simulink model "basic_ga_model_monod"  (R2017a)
settings: Solver=ode45  StartTime=0  StopTime=30  MaxStep=0.001  RelTol=1e-6  AbsTol=1e-6  EnableMultiTasking=on
undefined symbols (not defined in the file or in its folder): GA0, K, K1, K2, K3, Kga, Muga, Mumax, O20, S0, X0

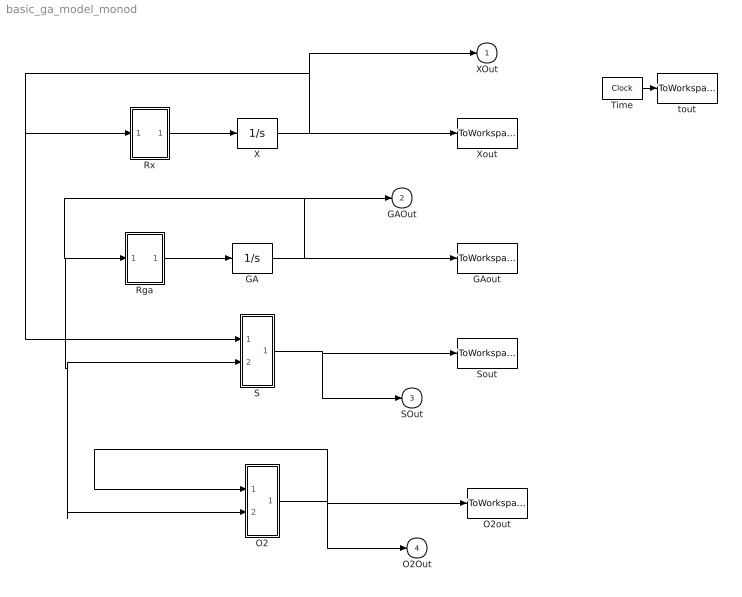
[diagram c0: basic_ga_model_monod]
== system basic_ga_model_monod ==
  GA : Integrator  InitialCondition=GA0  UpperSaturationLimit=1000  LowerSaturationLimit=0
  GAout : ToWorkspace  VariableName=GAout  SampleTime=-1
  O2 : Subsystem
  O2out : ToWorkspace  VariableName=O2out  SampleTime=-1
  Rga : Subsystem
  Rx : Subsystem
  S : Subsystem
  Sout : ToWorkspace  VariableName=Sout  SampleTime=-1
  Time : Clock
  X : Integrator  InitialCondition=X0  UpperSaturationLimit=1000  LowerSaturationLimit=0
  Xout : ToWorkspace  VariableName=Xout  SampleTime=-1
  tout : ToWorkspace  VariableName=tout  SampleTime=-1
  XOut : Outport
  GAOut : Outport  Port=2
  SOut : Outport  Port=3
  O2Out : Outport  Port=4
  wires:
  S/1(Sout) -> SOut/1, Sout/1
  Time/1 -> tout/1
  Rx/1(Rx) -> X/1
  Rga/1(Rga) -> GA/1
  GA/1 -> GAOut/1, O2/2(Rga), S/2(Rga), Rga/1(GA), GAout/1
  X/1 -> Xout/1, XOut/1, Rx/1(X), S/1(Rx)
  O2/1(O2out) -> O2/1(O2), O2Out/1, O2out/1

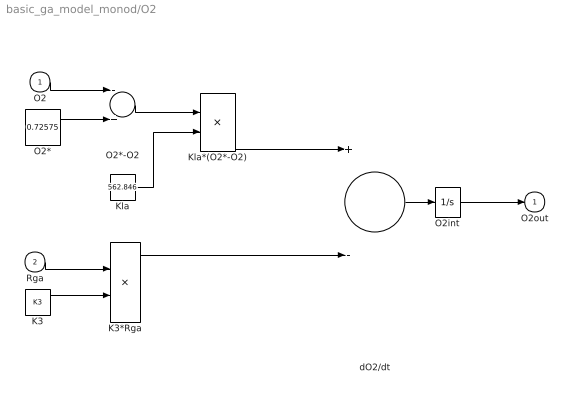
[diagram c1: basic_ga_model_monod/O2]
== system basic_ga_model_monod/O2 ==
  O2 : Inport
  Rga : Inport  Port=2
  K3 : Constant  Value=K3
  K3*Rga : Product
  Kla : Constant  Value=562.846
  Kla*(O2*-O2) : Product
  O2* : Constant  Value=0.72575
  O2*-O2 : Sum  Inputs=-+
  O2int : Integrator  InitialCondition=O20  UpperSaturationLimit=1000  LowerSaturationLimit=0
  dO2/dt : Sum  Inputs=+-
  O2out : Outport
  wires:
  O2int/1 -> O2out/1
  O2/1 -> O2*-O2/1
  K3*Rga/1 -> dO2/dt/2
  dO2/dt/1 -> O2int/1
  O2*/1 -> O2*-O2/2
  Rga/1 -> K3*Rga/1
  K3/1 -> K3*Rga/2
  O2*-O2/1 -> Kla*(O2*-O2)/1
  Kla/1 -> Kla*(O2*-O2)/2
  Kla*(O2*-O2)/1 -> dO2/dt/1

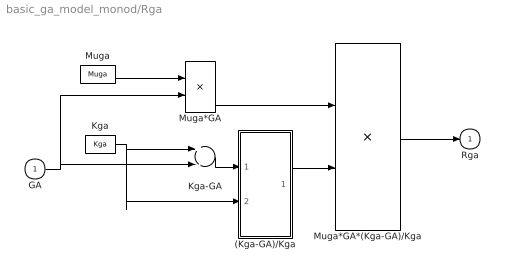
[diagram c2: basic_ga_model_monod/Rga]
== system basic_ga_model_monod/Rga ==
  GA : Inport
  (Kga-GA)/Kga : Subsystem
  Kga : Constant  Value=Kga
  Kga-GA : Sum  Inputs=+-
  Muga : Constant  Value=Muga
  Muga*GA : Product
  Muga*GA*(Kga-GA)/Kga : Product
  Rga : Outport
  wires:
  Muga*GA*(Kga-GA)/Kga/1 -> Rga/1
  Muga/1 -> Muga*GA/1
  Muga*GA/1 -> Muga*GA*(Kga-GA)/Kga/1
  GA/1 -> Kga-GA/2, Muga*GA/2
  Kga/1 -> (Kga-GA)/Kga/2(Ks+S), Kga-GA/1
  Kga-GA/1 -> (Kga-GA)/Kga/1(Mmax*S)
  (Kga-GA)/Kga/1(out_1) -> Muga*GA*(Kga-GA)/Kga/2

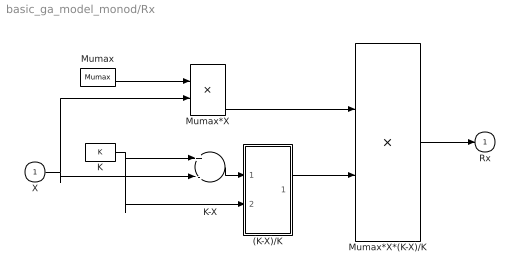
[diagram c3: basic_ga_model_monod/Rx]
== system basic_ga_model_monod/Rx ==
  X : Inport
  (K-X)/K : Subsystem
  K : Constant  Value=K
  K-X : Sum  Inputs=+-
  Mumax : Constant  Value=Mumax
  Mumax*X : Product
  Mumax*X*(K-X)/K : Product
  Rx : Outport
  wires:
  Mumax*X*(K-X)/K/1 -> Rx/1
  Mumax/1 -> Mumax*X/1
  Mumax*X/1 -> Mumax*X*(K-X)/K/1
  X/1 -> K-X/2, Mumax*X/2
  K/1 -> K-X/1, (K-X)/K/2(Ks+S)
  K-X/1 -> (K-X)/K/1(Mmax*S)
  (K-X)/K/1(out_1) -> Mumax*X*(K-X)/K/2

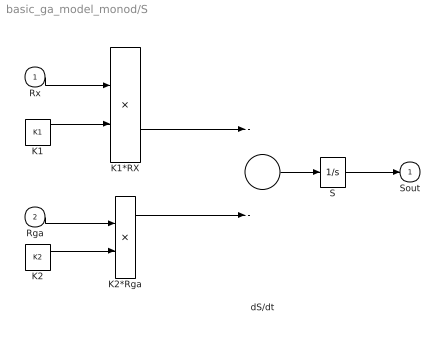
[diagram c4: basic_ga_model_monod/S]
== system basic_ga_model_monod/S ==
  Rx : Inport
  Rga : Inport  Port=2
  K1 : Constant  Value=K1
  K1*RX : Product
  K2 : Constant  Value=K2
  K2*Rga : Product
  S : Integrator  InitialCondition=S0  UpperSaturationLimit=1000  LowerSaturationLimit=0
  dS/dt : Sum  Inputs=--
  Sout : Outport
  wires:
  S/1 -> Sout/1
  Rx/1 -> K1*RX/1
  K1*RX/1 -> dS/dt/1
  K2*Rga/1 -> dS/dt/2
  dS/dt/1 -> S/1
  K1/1 -> K1*RX/2
  Rga/1 -> K2*Rga/1
  K2/1 -> K2*Rga/2

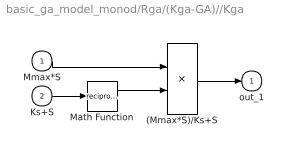
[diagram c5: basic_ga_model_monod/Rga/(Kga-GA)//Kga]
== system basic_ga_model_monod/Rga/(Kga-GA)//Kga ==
  Mmax*S : Inport
  Ks+S : Inport  Port=2
  (Mmax*S)/Ks+S : Product
  Math Function : Math  Operator=reciprocal
  out_1 : Outport
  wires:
  Mmax*S/1 -> (Mmax*S)/Ks+S/1
  Ks+S/1 -> Math Function/1
  Math Function/1 -> (Mmax*S)/Ks+S/2
  (Mmax*S)/Ks+S/1 -> out_1/1

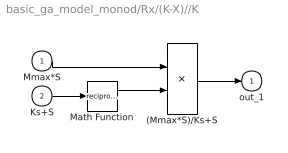
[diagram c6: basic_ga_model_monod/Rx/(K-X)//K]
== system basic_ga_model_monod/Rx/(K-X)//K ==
  Mmax*S : Inport
  Ks+S : Inport  Port=2
  (Mmax*S)/Ks+S : Product
  Math Function : Math  Operator=reciprocal
  out_1 : Outport
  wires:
  Mmax*S/1 -> (Mmax*S)/Ks+S/1
  Ks+S/1 -> Math Function/1
  Math Function/1 -> (Mmax*S)/Ks+S/2
  (Mmax*S)/Ks+S/1 -> out_1/1
